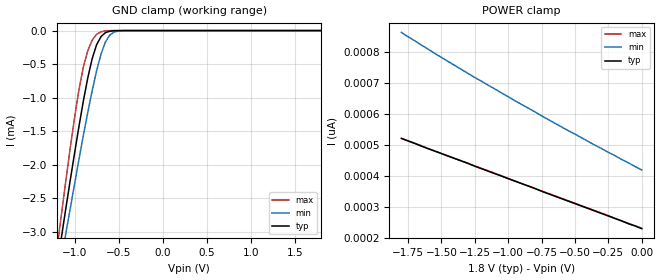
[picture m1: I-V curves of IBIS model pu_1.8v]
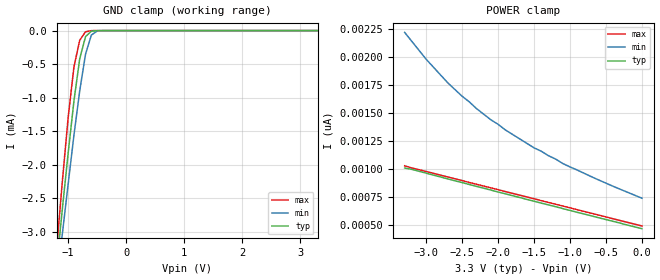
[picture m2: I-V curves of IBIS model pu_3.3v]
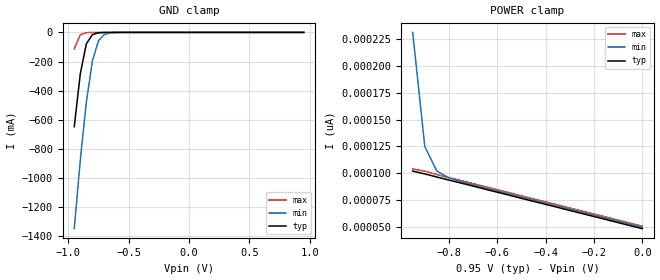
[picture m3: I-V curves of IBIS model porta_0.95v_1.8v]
|   DIODES CORP
|   IBIS Model of PI4ULS5V108
|   Product Family: ULS
|   TSSOP (L-20PIN) Package
[IBIS Ver] 4.0
[Comment char] |_char
[File Name] pi4uls5v108_l_revb.ibs
[File Rev] 2.0
[Source] File originated at Diodes Corp.
[Date] 04/09/20
[Disclaimer] (C) Copyright Diodes Corporation
   All rights reserved
  Diodes Semiconductor Corporation hereby grants the user of
  this IBIS model a non-exclusive, nontransferable license to
  use this IBIS model under the following terms.
  This IBIS model is provided on an "AS IS" basis and DIODES
  makes absolutely no warranty with respect to the information
  contained herein. DIODES DISCLAIMS AND CUSTOMER WAIVES ALL
  WARRANTIES, EXPRESSED OR IMPLIED, INCLUDING WARRANTIES OF
  MERCHANTABILITY OR FITNESS FOR A PARTICULAR PURPOSE. The
  entire risk as to quality and performance is with the customer.
  Accordingly, in no event shall the company be liable for any
  damages, whether in contract or tort, including any lost
  profits or other incidental, consequential, exemplary, or
  punitive damages arising out of the use or application of the
  IBIS model provided in this package. Further, DIODES reserves
  the right to make changes without notice to any product herein
  to improve reliability, function, or design. DIODES does not
  convey any license under patent rights or any other intellectual
  property rights, including those of third parties.
  The user is granted this license only to use the IBIS model
  and is not granted rights to sell, load, rent, lease or license
  the IBIS model in whole or in part, or in modified form to anyone
  other than user. User may modify the IBIS model to suit its specific
  application but rights to derivative works and such modifications
  shall belong to DIODES.
  Diodes is not obligated to provide maintenance or support
  for the licensed IBIS model.
  Contact DIODES at ATTN: APPLICATION ENGINEERING / IBIS MODELS
  1545 Barber Lane Milpitas, CA 95035 USA.
[Component] PI4ULS5V108
[Manufacturer] Diodes Corp.
[Package]
| Variable   typ   min   max
R_pkg   0.03869ohm   0.03668ohm   0.04069ohm
L_pkg   2.64482nH   2.06962nH   3.22001nH
C_pkg   0.19279pF   0.15543pF   0.23014pF
[Pin]  signal_name   model_name   R_pin   L_pin   C_pin
1   GND   GND   0.04069   3.22001nH   0.23014pF
2   VREFA   POWER   0.03969   2.93241nH   0.21146pF
3   A1   IO_A   0.03869   2.64482nH   0.19279pF
4   A2   IO_A   0.03768   2.35722nH   0.17411pF
5   A3   IO_A   0.03668   2.06962nH   0.15543pF
6   A4   IO_A   0.03668   2.06962nH   0.15543pF
7   A5   IO_A   0.03768   2.35722nH   0.17411pF
8   A6   IO_A   0.03869   2.64482nH   0.19279pF
9   A7   IO_A   0.03969   2.93241nH   0.21146pF
10   A8   IO_A   0.04069   3.22001nH   0.23014pF
11   B8   IO_B   0.04069   3.22001nH   0.23014pF
12   B7   IO_B   0.03969   2.93241nH   0.21146pF
13   B6   IO_B   0.03869   2.64482nH   0.19279pF
14   B5   IO_B   0.03768   2.35722nH   0.17411pF
15   B4   IO_B   0.03668   2.06962nH   0.15543pF
16   B3   IO_B   0.03668   2.06962nH   0.15543pF
17   B2   IO_B   0.03768   2.35722nH   0.17411pF
18   B1   IO_B   0.03869   2.64482nH   0.19279pF
19   VREFB   POWER   0.03969   2.93241nH   0.21146pF
20   EN   INPUT   0.04069   3.22001nH   0.23014pF
[Series Pin Mapping]   pin_2   model_name   function_table_group
3   18   mosfet   1
4   17   mosfet   1
5   16   mosfet   1
6   15   mosfet   1
7   14   mosfet   1
8   13   mosfet   1
9   12   mosfet   1
10   11   mosfet   1
[Series Switch Groups]
On 1 /
Off 1 /
[Model selector] INPUT
pu_1.8v   input pin w/int pu,vrefb=1.8v
pu_3.3v   input pin w/int pu,vrefb=3.3v
[Model selector] mosfet
mosfet_0.95v_1.8v  open drain io,vrefa=0.95v,vrefb=1.8v
mosfet_1.8v_3.3v   open drain io,vrefa=1.8v,vrefb=3.3v
[Model selector] IO_A
porta_0.95v_1.8v  open drain io,vrefa=0.95v,vrefb=1.8v
porta_1.8v_3.3v   open drain io,vrefa=1.8v,vrefb=3.3v
[Model selector] IO_B
portb_0.95v_1.8v  open drain io,vrefa=0.95v,vrefb=1.8v
portb_1.8v_3.3v   open drain io,vrefa=1.8v,vrefb=3.3v
[model] mosfet_1.8v_3.3v
Model_type Series_switch
Polarity   Non-Inverting
Enable   Active-High
| variable   typ   min   max
C_comp   9.837p   9.763p   9.906p
| variable   typ   min   max
[Voltage Range]   3.3V   3.3V   3.3V
[On]
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[Off]
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[model] mosfet_0.95v_1.8v
Model_type Series_switch
Polarity   Non-Inverting
Enable   Active-High
| variable   typ   min   max
C_comp   9.901p   9.824p   9.974p
| variable   typ   min   max
[Voltage Range]   1.8V   1.8V   1.8V
[On]
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[Off]
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| Models and submodels in the file (8): pu_1.8v (Input), pu_3.3v (Input), porta_0.95v_1.8v (Terminator), porta_1.8v_3.3v (Terminator), portb_0.95v_1.8v (Terminator), portb_1.8v_3.3v (Terminator), mosfet_1.8v_3.3v (Series_switch), mosfet_0.95v_1.8v (Series_switch)
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|   Model INPUT
[Model] pu_1.8v
Model_type Input
Vinl = 750.000mV
Vinh = 1.75000V
| variable   typ   min   max
C_comp   4.208pF   4.181pF   4.247pF
[Voltage Range]   1.8000V   1.6200V   1.9800V
[POWER Clamp Reference]   1.8000V   1.6200V   1.9800V
[GND Clamp Reference]   0.0000V   0.0000V   0.0000V
[Temperature Range]   25   85   -40
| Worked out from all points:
|   GND clamp passes 1 mA (typ) near -0.89 V on its own axis
[GND Clamp]
| Voltage   I(typ)   I(min)   I(max)
-1.8V     -8.89mA    -8.51mA    -9.73mA
-1.2V     -3.52mA    -3.8mA     -3.27mA
-1.15V    -3.09mA    -3.41mA    -2.75mA
-1.1V     -2.66mA    -3.03mA    -2.25mA
-1V       -1.83mA    -2.29mA    -1.3mA
-900mV    -1.05mA    -1.56mA    -543uA
-850mV    -706uA     -1.22mA    -302uA
-750mV    -212uA     -601uA     -55.5uA
-650mV    -31.3uA    -171uA     -4.68uA
-600mV    -9.33uA    -67.6uA    -1.03uA
-500mV    -666nA     -6.42uA    -31.3nA
1.8V      229pA      460pA      13.9pA
[POWER Clamp]
| Voltage   I(typ)   I(min)   I(max)
-1.8V     521pA      864pA      521pA
-1.55V    480pA      796pA      480pA
-1.25V    431pA      718pA      432pA
-950mV    383pA      643pA      383pA
-550mV    318pA      546pA      319pA
0V        229pA      419pA      230pA
[Model] pu_3.3v
Model_type Input
Vinl = 990.000mV
Vinh = 2.31000V
| variable   typ   min   max
C_comp   4.148pF   4.123pF   4.187pF
[Voltage Range]   3.3000V   3.0000V   3.6000V
[POWER Clamp Reference] 3.3000V   3.0000V   3.6000V
[GND Clamp Reference]   0.0000V   0.0000V   0.0000V
[Temperature Range]   25   85   -40
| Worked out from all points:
|   GND clamp passes 1 mA (typ) near -0.89 V on its own axis
[GND Clamp]
| Voltage   I(typ)   I(min)   I(max)
-3.3V     -22.4mA    -20.3mA    -26mA
-1.2V     -3.52mA    -3.8mA     -3.27mA
-1.1V     -2.66mA    -3.03mA    -2.25mA
-1V       -1.83mA    -2.29mA    -1.3mA
-900mV    -1.05mA    -1.56mA    -543uA
-800mV    -419uA     -897uA     -143uA
-700mV    -90.5uA    -352uA     -17.8uA
-600mV    -9.33uA    -67.6uA    -1.03uA
-500mV    -666nA     -6.42uA    -31.3nA
3.3V      469pA      828pA      439pA
[POWER Clamp]
| Voltage   I(typ)   I(min)   I(max)
-3.3V     1.01nA     2.22nA     1.03nA
-3V       964pA      1.98nA     979pA
-2.7V     913pA      1.77nA     930pA
-2.5V     880pA      1.65nA     898pA
-2.4V     863pA      1.6nA      881pA
-2.3V     846pA      1.54nA     865pA
-2.1V     813pA      1.44nA     833pA
-1.9V     780pA      1.35nA     800pA
-1.5V     714pA      1.19nA     736pA
-1.1V     648pA      1.05nA     671pA
-600mV    566pA      903pA      590pA
0V        469pA      741pA      493pA
|   Model IO_A
[Model]   porta_0.95v_1.8v
Model_type Terminator
| variable   typ   min   max
C_comp   3.5561p   3.5280p   3.5829p
[Voltage Range]   0.9500V   0.9000V   1.0000V
[POWER Clamp Reference]   0.9500V   0.9000V   1.0000V
[GND Clamp Reference]   0.0000V   0.0000V   0.0000V
[Temperature Range]   25   85   -40
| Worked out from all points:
|   GND clamp passes 1 mA (typ) near -0.71 V on its own axis
[GND Clamp]
| Voltage   I(typ)   I(min)   I(max)
-950mV    -647.9mA   -1.348A    -112.9mA
-900mV    -283.7mA   -877.9mA   -15.94mA
-850mV    -78.75mA   -479.3mA   -1.974mA
-800mV    -15.25mA   -197mA     -233.3uA
-750mV    -2.808mA   -57.58mA   -23.15uA
-700mV    -522.2uA   -13.76mA   -2.027uA
-650mV    -90.53uA   -3.186mA   -172.5nA
-550mV    -2.164uA   -174uA     -1.291nA
950mV     48.47pA    52.46pA    47.94pA
[POWER Clamp]
| Voltage   I(typ)   I(min)   I(max)
-950mV    102pA      231pA      104pA
-900mV    99.4pA     125pA      102pA
-850mV    96.5pA     102pA      98.8pA
-800mV    93.7pA     95.7pA     96pA
-750mV    90.9pA     92.2pA     93.2pA
0V        48.5pA     49.6pA     50.8pA
